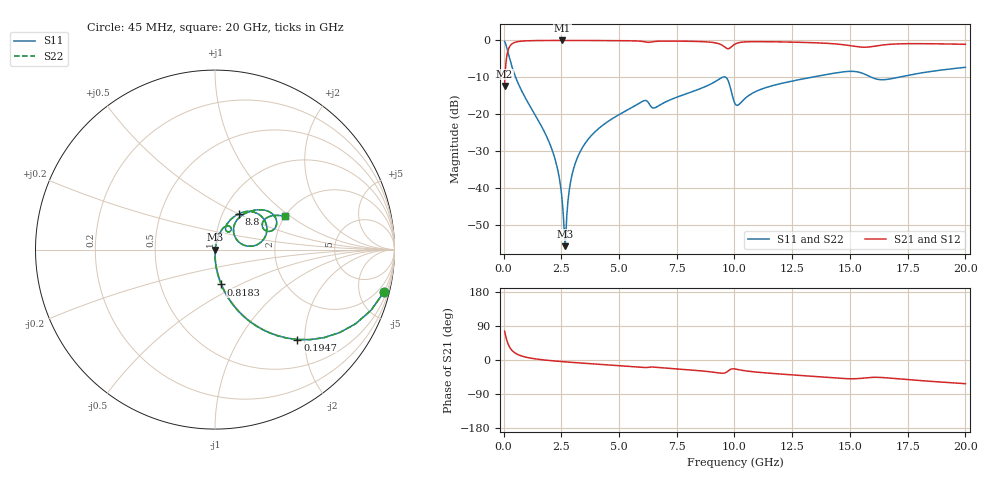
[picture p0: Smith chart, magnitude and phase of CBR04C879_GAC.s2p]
! S-parameter model data by Modelithics Inc.  support@modelithics.com 813-866-6335  Tampa FL USA
! S-Parameter data specifications:
! Substrate: 20-mil Rogers 4350B, substrate thickness, H=0.508mm, Dielectric constant, Er=3.75
! PCB Mounting Pad Footprint: Pad width, PadW=0.52mm , Pad length, PadL=0.52mm , Pad gap, PadG (edge-to-edge)=0.28mm , Reference planes=1.32mm apart
#  GHz  S  MA  R 50
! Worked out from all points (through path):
!   801 points, 45 MHz to 20 GHz, reference 50 ohm
!   highest |S21| = -0.01 dB at 2.539 GHz (marker M1); lowest = -12.4 dB at 45 MHz (marker M2)
!   group delay of S21, straight-line fit = 9.92 ps
!   lowest |S11| = -55.8 dB at 2.664 GHz (marker M3), VSWR 1.00, Z = 50.2 - j0.00597 ohm
!   |S11| at or under -10 dB: 523.6 MHz to 9.479 GHz (8.956 GHz wide, 179 % of centre); 9.621 GHz to 13.33 GHz (3.713 GHz wide, 32.4 % of centre); 15.93 GHz to 17.09 GHz (1.164 GHz wide, 7.05 % of centre)
!   |S22| runs from -55.8 to -0.3 dB; largest |S21 - S12| = 0
!   S11 on the Smith chart (normalised r, x): 45 MHz: 0.99, -8.02; 194.7 MHz: 0.99, -1.84; 818.3 MHz: 0.99, -0.40; 8.8 GHz: 1.19, +0.51; 20 GHz: 2.00, +0.91
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0.045  0.9706 -14.0  0.2406 76.0  0.2406 76.0  0.9706 -14.0
0.194662  0.6799 -47.5  0.7329 42.5  0.7329 42.5  0.6799 -47.5
0.419156  0.389 -67.8  0.9206 22.1  0.9206 22.1  0.389 -67.8
0.818256  0.1971 -79.9  0.9795 9.9  0.9795 9.9  0.1971 -79.9
2.090387  0.03358 -89.5  0.9979 -1.9  0.9979 -1.9  0.03358 -89.5
2.364769  0.01645 -88.1  0.9983 -3.4  0.9983 -3.4  0.01645 -88.1
2.539375  0.006729 -80.7  0.9983 -4.3  0.9983 -4.3  0.006729 -80.7
2.664094  0.001621 -2.1  0.9983 -4.9  0.9983 -4.9  0.001621 -2.1
2.738925  0.004244 61.9  0.9983 -5.3  0.9983 -5.3  0.004244 61.9
2.8387  0.009038 73.6  0.9982 -5.7  0.9982 -5.7  0.009038 73.6
2.963419  0.01498 77.1  0.9981 -6.3  0.9981 -6.3  0.01498 77.1
3.387462  0.034 78.7  0.9974 -8.2  0.9974 -8.2  0.034 78.7
4.260494  0.06941 76.3  0.9952 -11.8  0.9952 -11.8  0.06941 76.3
5.956669  0.1456 64.5  0.9735 -19.3  0.9735 -19.3  0.1456 64.5
6.704981  0.1294 63.1  0.9753 -19.7  0.9753 -19.7  0.1294 63.1
8.800256  0.2412 56.2  0.9548 -30.1  0.9548 -30.1  0.2412 56.2
9.598456  0.3189 26.8  0.8038 -33.8  0.8038 -33.8  0.3189 26.8
10.0225  0.1388 18.0  0.8918 -23.7  0.8918 -23.7  0.1388 18.0
13.36496  0.3175 44.0  0.9318 -43.1  0.9318 -43.1  0.3175 44.0
15.26069  0.3773 24.4  0.8261 -49.3  0.8261 -49.3  0.3773 24.4
16.68248  0.2984 28.2  0.8831 -47.5  0.8831 -47.5  0.2984 28.2
20  0.4316 25.4  0.8854 -62.5  0.8854 -62.5  0.4316 25.4
